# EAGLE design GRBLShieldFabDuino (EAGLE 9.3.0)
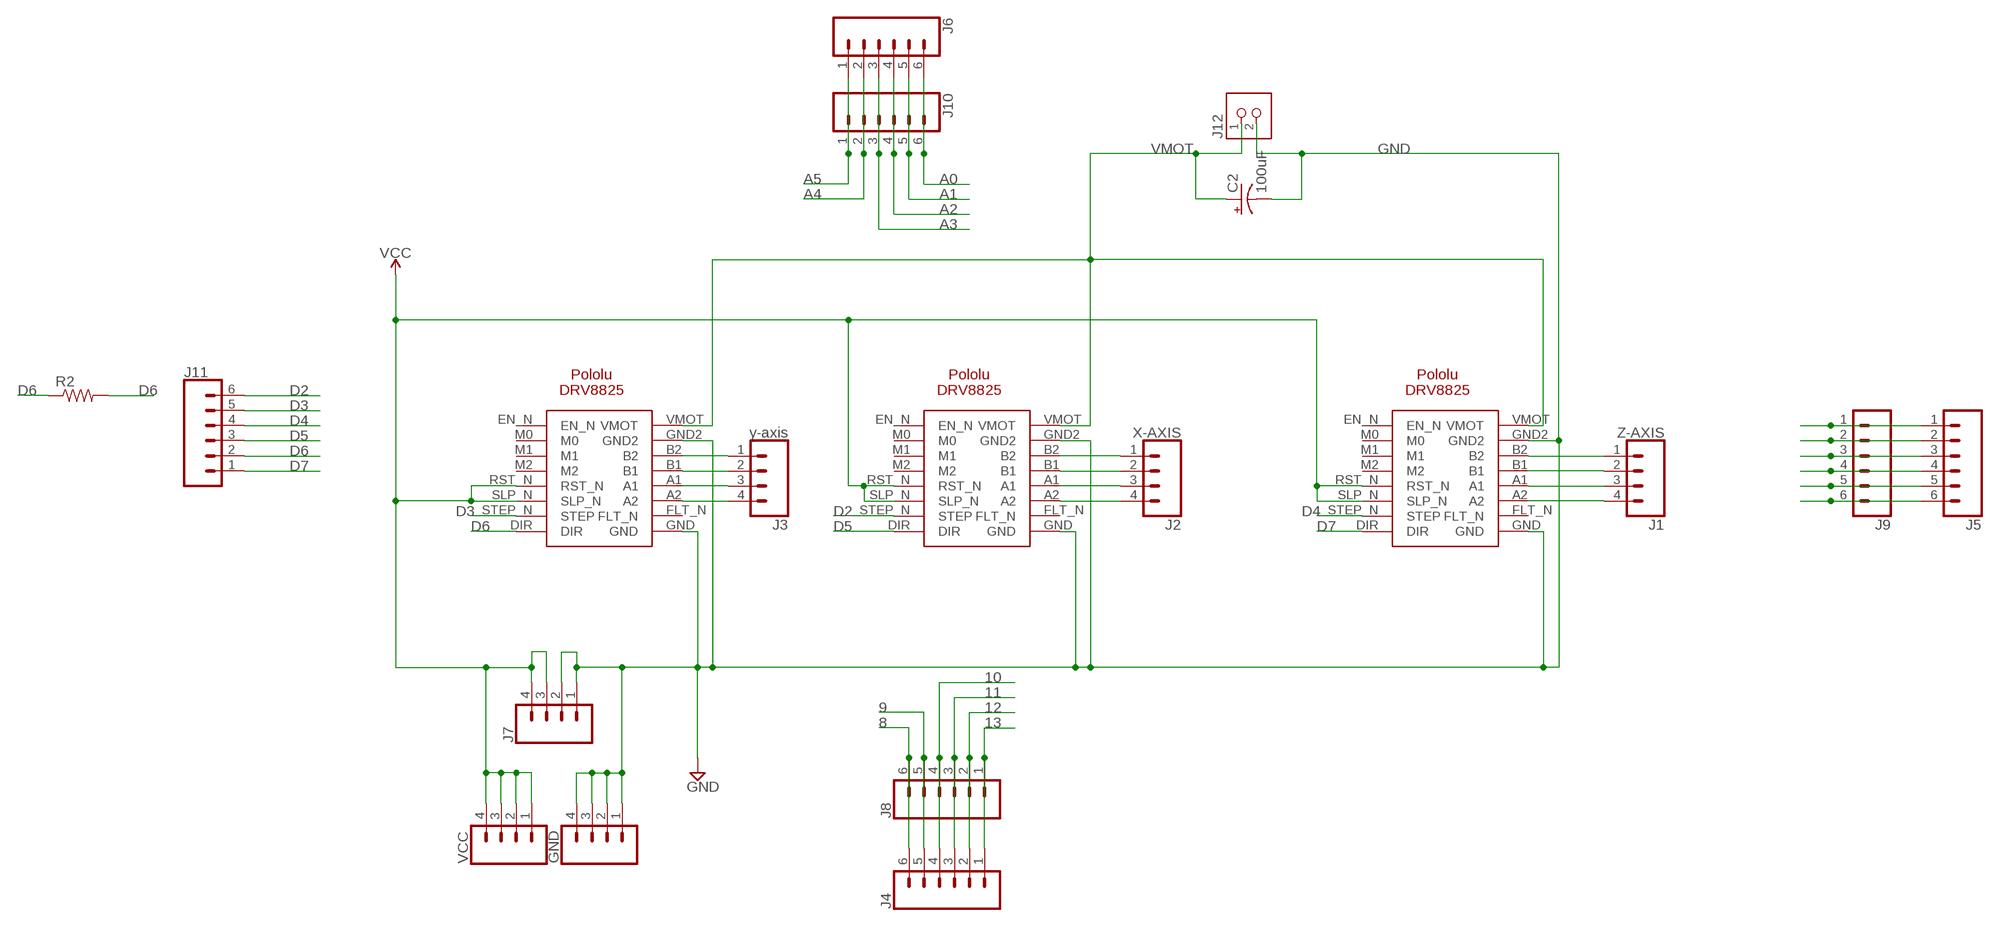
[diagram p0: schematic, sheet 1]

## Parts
C2  100uF  SPARKFUN-CAPACITORS_100UF-POLAR-RADIAL-2.5MM-25V-20%  [SPARKFUN-CAPACITORS_CPOL-RADIAL-2.5MM-6.5MM]
GND  CONN_04PTH  [1X04]
J1  Z-AXIS  CONN_04PTH  [1X04]
J2  X-AXIS  CONN_04PTH  [1X04]
J3  y-axis  CONN_04PTH  [1X04]
J4  CONN_06SILK_FEMALE_PTH  [1X06]
J5  CONN_06SILK_FEMALE_PTH  [1X06]
J6  CONN_06SILK_FEMALE_PTH  [1X06]
J7  SPARKFUN-CONNECTORS_CONN_04PTH  [SPARKFUN-CONNECTORS_1X04]
J8  CONN_06FEMALE_LOCK  [1X06_FEMALE_LOCK.010]
J9  CONN_06FEMALE_LOCK  [1X06_FEMALE_LOCK.010]
J10  CONN_06FEMALE_LOCK  [1X06_FEMALE_LOCK.010]
J11  CONN_06FEMALE_LOCK  [1X06_FEMALE_LOCK.010]
J12  FAB_TERM-1X02-ADAFRUIT  [FAB_3.5MMTERM]
R2  RES-US1206FAB  [R1206FAB]
VCC  CONN_04PTH  [1X04]
X  POLOLU-DRV8825  [POLOLU-DRV8825]
Y  POLOLU-DRV8825  [POLOLU-DRV8825]
Z  POLOLU-DRV8825  [POLOLU-DRV8825]

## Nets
8: J4.6 J8.6
9: J4.5 J8.5
10: J4.4 J8.4
11: J4.3 J8.3
12: J4.2 J8.2
13: J4.1 J8.1
A0: J6.6 J10.6
A1: J6.5 J10.5
A2: J6.4 J10.4
A3: J6.3 J10.3
A4: J6.2 J10.2
A5: J6.1 J10.1
D2: J11.6 X.STEP_N(STEP)
D3: J11.5 Y.STEP_N(STEP)
D4: J11.4 Z.STEP_N(STEP)
D5: J11.3 X.DIR
D6: J11.2 R2.1 R2.2 Y.DIR
D7: J11.1 Z.DIR
GND: C2.2(-) GND.1 GND.2 GND.3 GND.4 J7.1 J7.2 J12.2 X.GND X.GND2 Y.GND Y.GND2 Z.GND Z.GND2
N$1: J1.1 Z.B2
N$2: J1.2 Z.B1
N$3: J1.3 Z.A1
N$4: J1.4 Z.A2
N$5: J2.1 X.B2
N$6: J2.2 X.B1
N$7: J2.3 X.A1
N$8: J2.4 X.A2
N$9: J3.1 Y.B2
N$10: J3.2 Y.B1
N$11: J3.3 Y.A1
N$12: J3.4 Y.A2
N$13: J5.1 J9.1
N$14: J5.2 J9.2
N$15: J5.3 J9.3
N$16: J5.4 J9.4
N$17: J5.5 J9.5
N$18: J5.6 J9.6
VCC: J7.3 J7.4 VCC.1 VCC.2 VCC.3 VCC.4 X.RST_N X.SLP_N Y.RST_N Y.SLP_N Z.RST_N Z.SLP_N
VMOT: C2.1(+) J12.1 X.VMOT Y.VMOT Z.VMOT
Unconnected: X.EN_N X.FLT_N X.M0 X.M1 X.M2 Y.EN_N Y.FLT_N Y.M0 Y.M1 Y.M2 Z.EN_N Z.FLT_N Z.M0 Z.M1 Z.M2

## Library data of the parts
C2 = GRBLShieldFabDuino:SPARKFUN-CAPACITORS_100UF-POLAR: 100µF polarized capacitors; PROD_ID: CAP-08439
GND J1-J3 VCC = SparkFun-Connectors:CONN_04: Multi connection point. Often used as Generic Header-pin footprint for 0.1 inch spaced/style header connections On any of the 0.1 inch spaced packages, you can populate with these: Break Away Headers - Straight (PRT-00116) Break Away Male Headers - Right Angle (PRT-00553) Female Headers (PRT-00115)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; PROD_ID: CONN-09696
J4-J6 = SparkFun-Connectors:CONN_06: Multi connection point. Often used as Generic Header-pin footprint for 0.1 inch spaced/style header connections On any of the 0.1 inch spaced packages, you can populate with these: Break Away Headers - Straight (PRT-00116) Break Away Male Headers - Right Angle (PRT-00553) Female Headers (PRT-00115)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; PROD_ID: CONN-08437
J7 = GRBLShieldFabDuino:SPARKFUN-CONNECTORS_CONN_04: Multi connection point. Often used as Generic Header-pin footprint for 0.1 inch spaced/style header connections On any of the 0.1 inch spaced packages, you can populate with these: Break Away Headers - Straight (PRT-00116) Break Away Male Headers - Right Angle (PRT-00553) Female Headers (PRT-00115)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; PROD_ID: CONN-09696
J8-J11 = SparkFun-Connectors:CONN_06: Multi connection point. Often used as Generic Header-pin footprint for 0.1 inch spaced/style header connections On any of the 0.1 inch spaced packages, you can populate with these: Break Away Headers - Straight (PRT-00116) Break Away Male Headers - Right Angle (PRT-00553) Female Headers (PRT-00115)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
J12 = GRBLShieldFabDuino:FAB_TERM-1X02: 3.5mm terminal block, 2 positions ED555-2DS as found in the fablab inventory.
R2 = fab:RES-US: Resistor (US Symbol)
X Y Z = alvarop-lib:POLOLU-DRV8825

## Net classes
0 default: clearance 0.406 mm

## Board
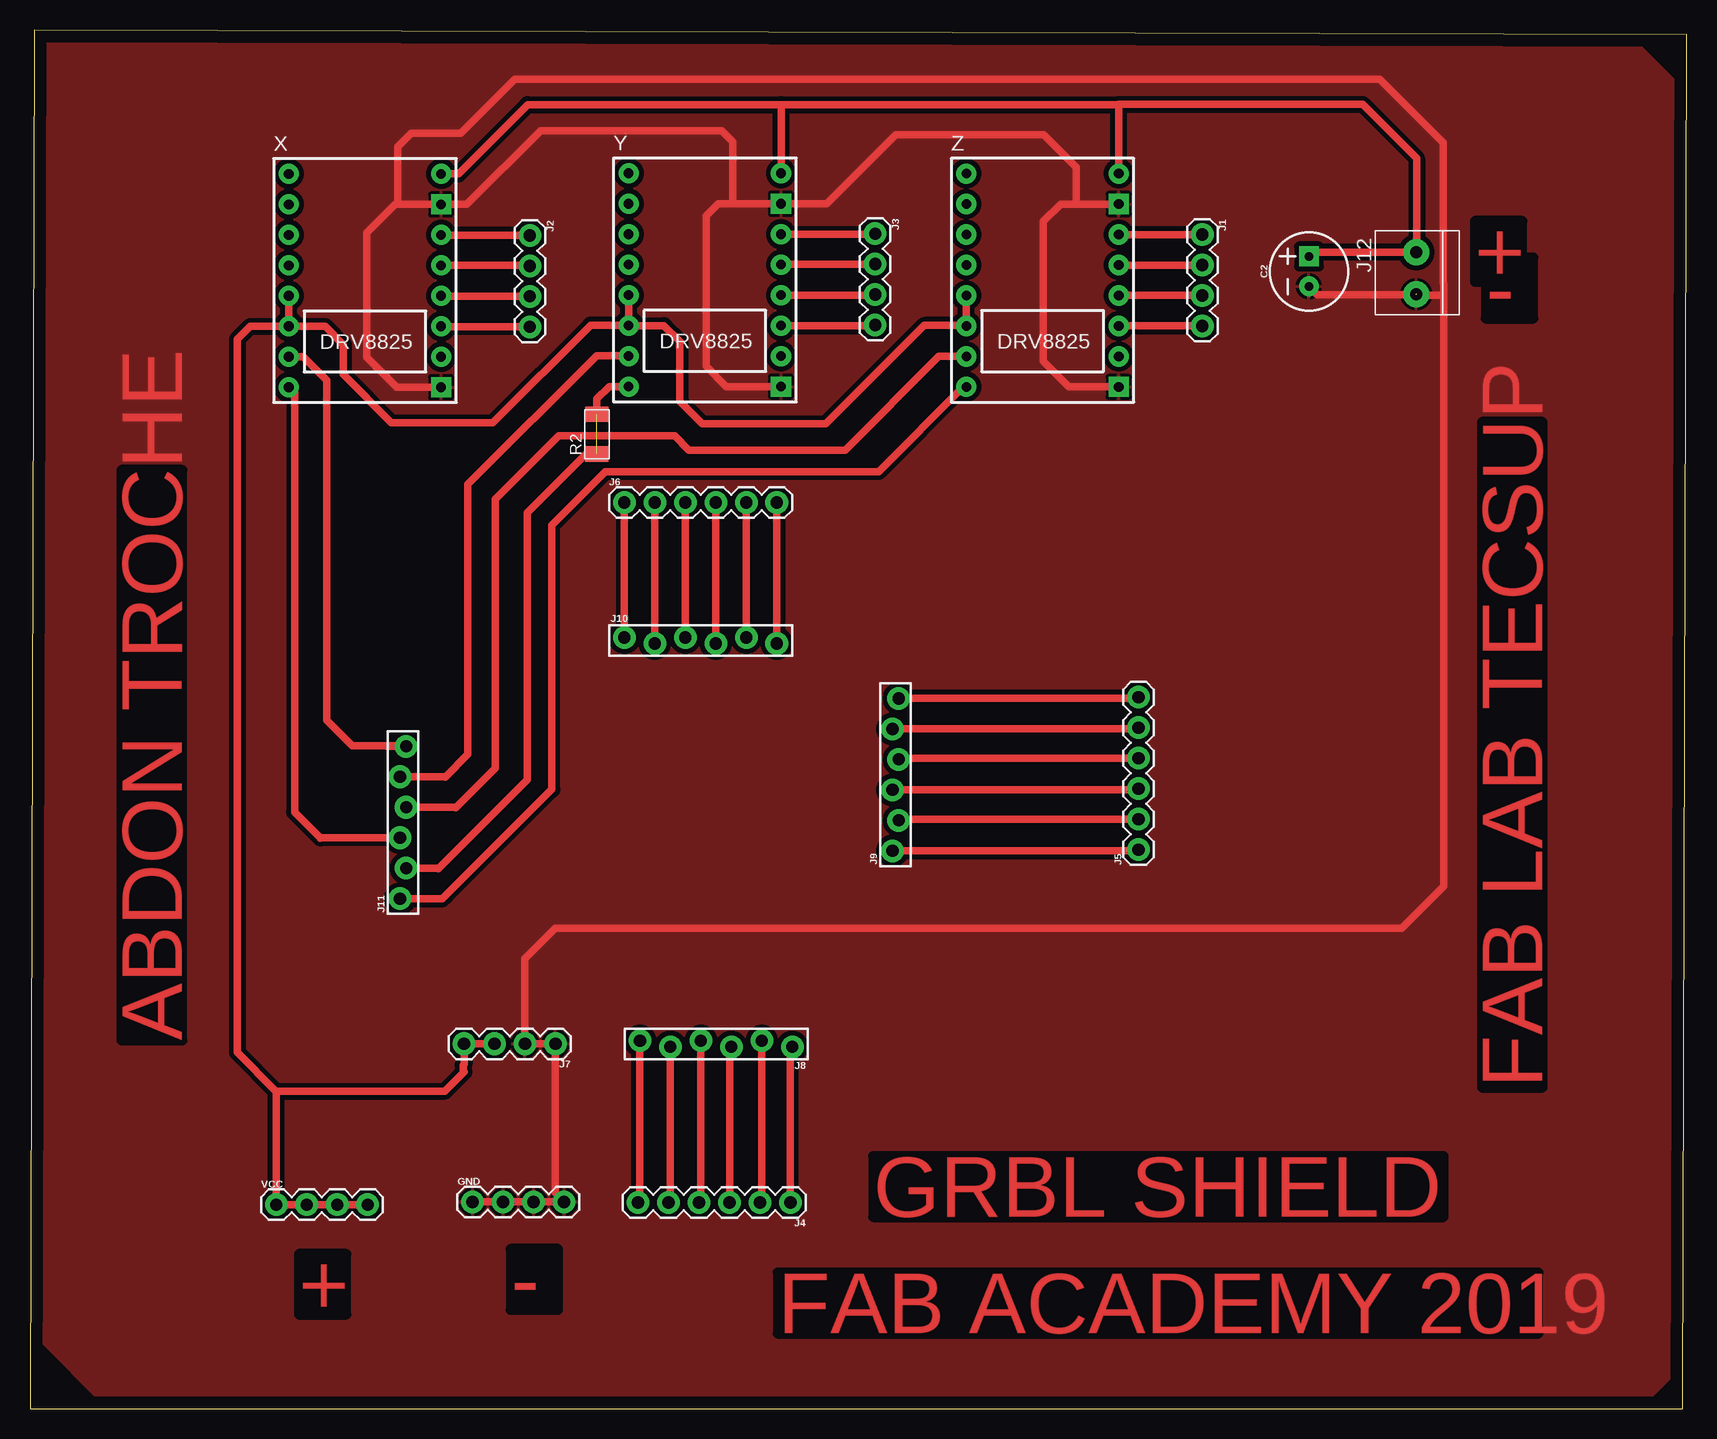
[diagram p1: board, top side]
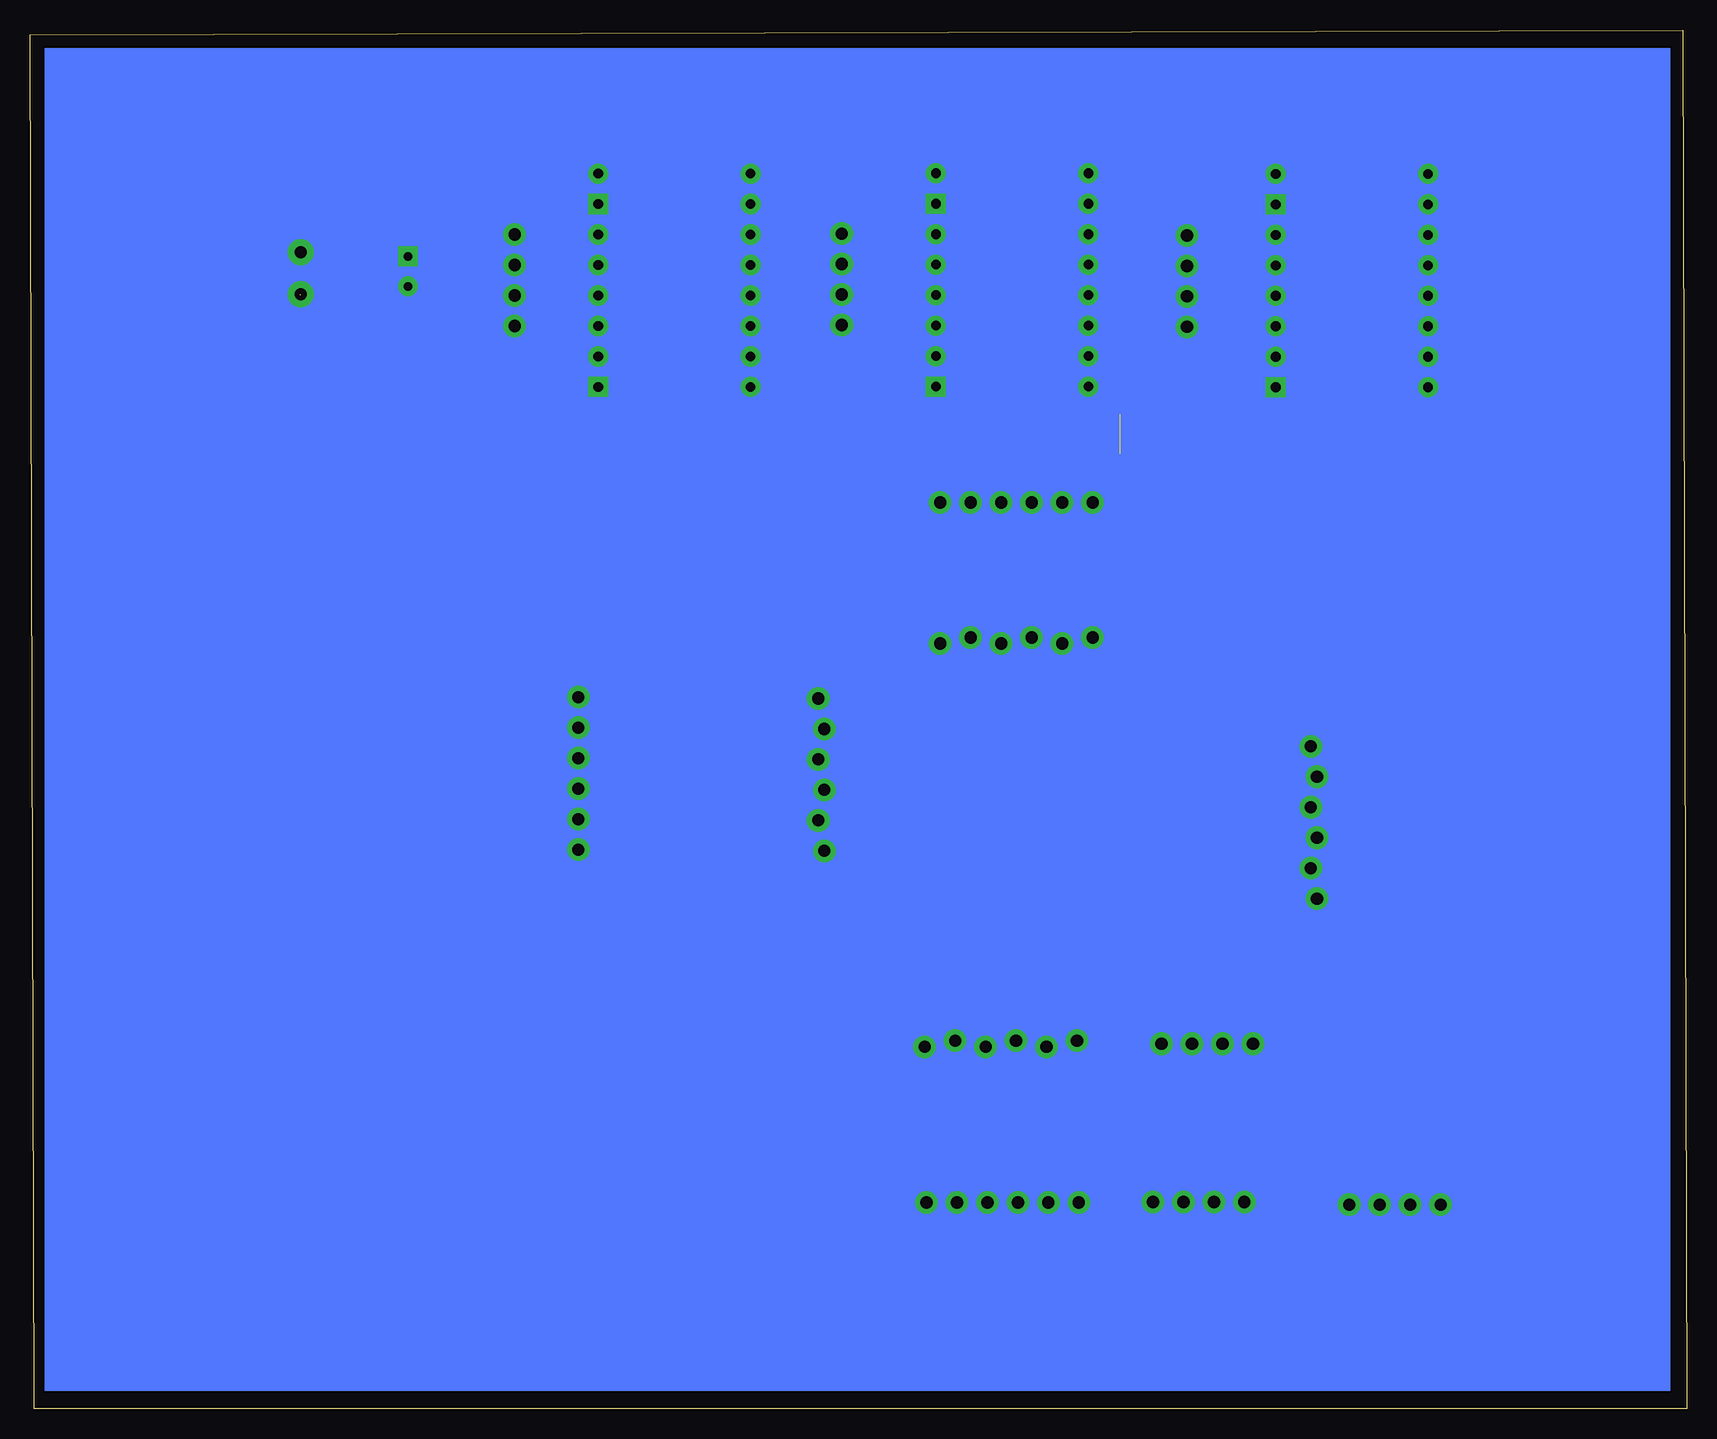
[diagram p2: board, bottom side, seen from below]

Size 138.08 x 114.91 mm. Coordinates in mm from the lower left corner, seen from the top.
Outline: 0,0 137.72,0.03 138.08,114.53 0.36,114.91 0,0
Copper layers (1*16): Top 0.035mm / dielectric 1.5mm / Bottom 0.035mm
Design rules "default": minimum track width 6mil, minimum drill 0.35mm, track to track 6mil, track to pad 6mil, pad to pad 6mil, via to via 6mil, smd to smd 6mil, copper to edge 40mil, drill to drill 6mil, minimum pad ring 10mil, minimum via ring 8mil, stop-mask expansion 4mil, vias tented up to drill 0mil, thermal gap 10mil

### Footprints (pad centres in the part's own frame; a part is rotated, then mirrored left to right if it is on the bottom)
SPARKFUN-CAPACITORS_CPOL-RADIAL-2.5MM-6.5MM = drill 0.7 pad 1.651 square: 1 1.25,0 | drill 0.7 pad 1.651: 2 -1.25,0
1X04 = drill 1.016 pad 1.88: 1 0,0; 2 2.54,0; 3 5.08,0; 4 7.62,0
1X06 = drill 1.016 pad 1.88: 1 0,0; 2 2.54,0; 3 5.08,0; 4 7.62,0; 5 10.16,0; 6 12.7,0
SPARKFUN-CONNECTORS_1X04 = drill 1.016 pad 1.88: 1 0,0; 2 2.54,0; 3 5.08,0; 4 7.62,0
1X06_FEMALE_LOCK.010 = drill 1.016 pad 1.88: 1 0,0.254; 2 2.54,-0.254; 3 5.08,0.254; 4 7.62,-0.254; 5 10.16,0.254; 6 12.7,-0.254
FAB_3.5MMTERM = drill 1 pad 2.184: 1 1.8,0; 2 -1.7,0
R1206FAB = smd 1.27 x 1.905: 1 -1.651,0; 2 1.651,0
POLOLU-DRV8825 = drill 0.8 pad 1.676: A1 6.35,-1.27; A2 6.35,-3.81; B1 6.35,1.27; B2 6.35,3.81; DIR -6.35,-8.89; EN_N -6.35,8.89; FLT_N 6.35,-6.35; M0 -6.35,6.35; M1 -6.35,3.81; M2 -6.35,1.27; RST_N -6.35,-1.27; SLP_N -6.35,-3.81; STEP_N -6.35,-6.35; VMOT 6.35,8.89 | drill 0.8 pad 1.676 square: GND 6.35,-8.89; GND2 6.35,6.35

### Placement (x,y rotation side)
C2  106.58,94.79 90 top
GND  36.88,17.25 0 top
J1  97.69,97.87 270 top
J2  41.66,97.79 270 top
J3  70.43,97.94 270 top
J4  63.37,17.2 180 top
J5  92.38,46.61 90 top
J6  49.53,75.54 0 top
J7  43.79,30.43 180 top
J8  63.53,30.43 180 top
J9  72.14,46.51 90 top
J10  49.53,64.03 0 top
J11  31.09,42.52 90 top
J12  115.52,94.59 90 top
R2  47.24,81.23 90 top
VCC  20.52,17.02 0 top
X  27.91,94.03 0 top
Y  56.24,94.08 0 top
Z  84.38,94.06 0 top

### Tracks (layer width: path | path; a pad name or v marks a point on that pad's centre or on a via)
8
  Top 0.61: J4.6 50.83,17.35 J8.6
9
  Top 0.61: J8.5 53.37,17.35 J4.5
10
  Top 0.61: J8.4 55.91,17.35 J4.4
11
  Top 0.61: J4.3 58.29,30.02 J8.3
12
  Top 0.61: J8.2 60.99,17.6 61.39,17.2 61.39,17.3 61.29,17.2 J4.2
13
  Top 0.61: J4.1 63.37,30.02 J8.1
A0
  Top 0.61: J6.6 J10.6
A1
  Top 0.61: J6.5 J10.5
A2
  Top 0.61: J10.4 J6.4
A3
  Top 0.61: J6.3 J10.3
A4
  Top 0.61: J10.2 J6.2
A5
  Top 0.61: J6.1 J10.1
D2
  Top 0.61: 29.67,55.25 26.87,55.25 24.74,57.38 24.74,85.73 22.78,87.68 X.STEP_N | 29.67,55.25 31.04,55.25 | J11.6 29.69,55.22 29.67,55.25
D3
  Top 0.61: Y.STEP_N 49.86,87.76 47.22,87.76 36.5,77.04 36.5,54.56 34.59,52.65 34.57,52.68 J11.5
D4
  Top 0.61: Z.STEP_N 75.74,87.71 67.94,79.91 54.89,79.91 53.72,81.08 44.04,81.08 38.76,75.79 38.76,53.39 35.48,50.11 35.46,50.14 J11.4
D5
  Top 0.61: 24.18,47.6 24.21,47.57 | X.DIR 21.59,85.14 22.05,84.68 22.05,49.73 24.02,47.76 24.18,47.6 | J11.3 24.18,47.6
D6  (1 unrouted)
  Top 0.61: 34.06,45.06 34.04,45.03 | R2.2 47.24,84.18 48.26,85.19 Y.DIR | R2.1 46.35,79.58 41.45,74.68 41.45,52.45 34.3,45.3 34.06,45.06 | J11.2 34.06,45.06
D7
  Top 0.61: 34.34,42.49 34.37,42.52 | Z.DIR 77.77,85.17 70.71,78.11 47.95,78.11 43.48,73.63 43.48,51.64 34.61,42.76 34.37,42.52 | J11.1 34.37,42.52
GND  (1 unrouted)
  Top 0.61: 58.57,100.43 57.35,100.43 56.34,99.42 56.34,86.89 58.04,85.19 Y.GND | 87.2,100.41 85.88,100.41 84.43,98.96 84.43,87.3 86.56,85.17 Z.GND | 30.63,100.38 30.43,100.38 28.07,98.02 28.07,87.66 30.58,85.14 X.GND | 30.63,100.38 30.63,105.18 31.78,106.32 35.92,106.32 40.41,110.82 112.47,110.82 117.78,105.51 117.78,93.79 117.8,93.76 117.8,92.81 | 117.8,92.81 117.8,43.56 114.3,40.06 43.79,40.06 41.25,37.52 J7.2 J7.1 43.79,18.01 44.5,17.3 GND.4 GND.3 GND.2 GND.1 | 117.8,92.81 117.78,92.84 | 58.57,100.43 58.57,105.61 57.66,106.53 42.54,106.53 36.4,100.38 X.GND2 30.63,100.38 | 87.2,100.41 87.2,103.48 84.48,106.2 72.16,106.2 66.4,100.43 Y.GND2 58.57,100.43 | 117.8,92.81 115.6,92.81 115.54,92.86 107.26,92.86 C2.2 | Z.GND2 87.2,100.41
  pour Top: 1.75,114.35 133.43,114.35 137.97,109.8 137.97,3.84 134.24,0.1 6.4,0.1 0.51,5.99 0.51,113.11
N$1
  Top 0.61: J1.1 Z.B2
N$2
  Top 0.61: Z.B1 J1.2
N$3
  Top 0.61: J1.3 Z.A1
N$4
  Top 0.61: Z.A2 J1.4
N$5
  Top 0.61: 41.6,97.84 J2.1 34.32,97.79 X.B2
N$6
  Top 0.61: J2.2 41.6,95.3 X.B1
N$7
  Top 0.61: 41.6,92.76 J2.3 34.32,92.71 X.A1
N$8
  Top 0.61: 41.6,90.22 J2.4 34.32,90.17 X.A2
N$9
  Top 0.61: Y.B2 70.38,97.89 J3.1
N$10
  Top 0.61: J3.2 62.64,95.4 Y.B1
N$11
  Top 0.61: J3.3 70.38,92.81 Y.A1
N$12
  Top 0.61: Y.A2 70.38,90.27 J3.4
N$13
  Top 0.61: J9.1 92.28,46.51 J5.1
N$14
  Top 0.61: J5.2 72.49,49.15 J9.2
N$15
  Top 0.61: J9.3 92.28,51.59 J5.3
N$16
  Top 0.61: J5.4 72.49,54.23 J9.4
N$17
  Top 0.61: J9.5 92.91,56.67 92.94,56.69 92.86,56.77 J5.5
N$18
  Top 0.61: J5.6 92.28,59.21 J9.6
VCC
  Top 0.61: 20.5,26.49 17.27,29.72 17.27,89.13 18.36,90.22 X.SLP_N | 20.5,26.49 34.57,26.49 36.17,28.09 36.09,28.17 36.09,28.65 36.17,28.73 J7.4 J7.3 | 20.57,26.42 20.52,26.47 | VCC.4 VCC.3 VCC.2 VCC.1 20.52,26.47 | 20.52,26.47 20.5,26.49 | Y.SLP_N Y.RST_N | Y.SLP_N 49.83,90.32 46.71,90.32 38.58,82.19 30.12,82.19 26.11,86.21 26.11,88.7 24.59,90.22 X.SLP_N | Y.SLP_N 52.83,90.27 54.13,88.98 54.13,83.97 56.01,82.09 66.32,82.09 74.52,90.3 77.98,90.3 Z.SLP_N Z.RST_N | X.SLP_N X.RST_N | X.SLP_N 21.69,90.09
VMOT
  Top 0.61: 62.59,108.69 41.48,108.69 35.71,102.92 X.VMOT | 90.73,108.69 90.73,108.71 111.05,108.71 115.54,104.22 115.54,96.42 J12.1 106.92,96.39 C2.1 106.9,96.36 | 62.59,108.69 90.73,108.69 | Y.VMOT 62.59,108.69 | Z.VMOT 90.73,108.69
(copper drawn outside any net)
  shapes: Bottom area x1

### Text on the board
Top: + | - | ABDON TROCHE | FAB LAB TECSUP | GRBL SHIELD | - | + | FAB ACADEMY 2019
